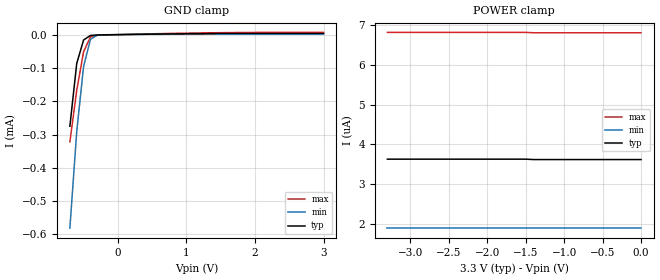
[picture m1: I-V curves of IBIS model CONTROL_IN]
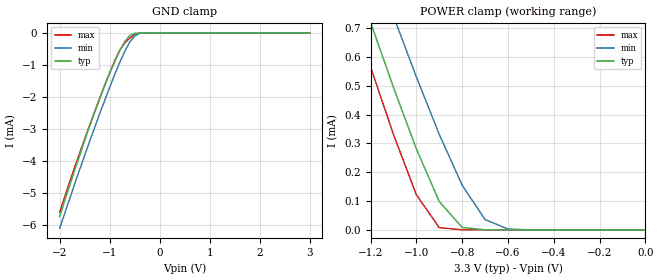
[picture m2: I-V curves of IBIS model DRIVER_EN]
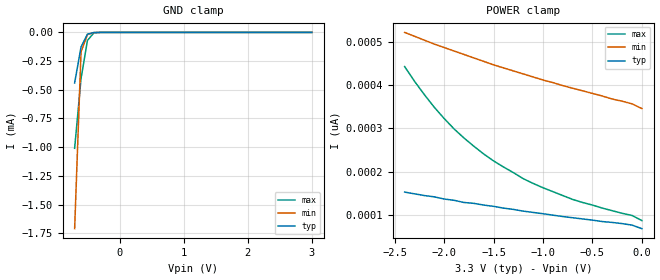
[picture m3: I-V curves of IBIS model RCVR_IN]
|   Texas Instruments Incorporated
|   Data Transmissions Products
|   IBIS Model for SN65LVDS122
|   16D SOIC Package
[IBIS Ver]   3.2
[Comment char]   |_char
[File name]   lvds122.ibs
[File Rev]   3.0
[Date]   22Sep03
[Source]   File originated at Texas Instruments Incorporated.
   Data Transmission Products Group.
[Notes]
[Disclaimer]
(C) Copyright Texas Instruments Incorporated 2002
   All rights reserved
  Texas Instruments Incorporated hereby grants the user of this IBIS
model a non-exclusive, nontransferable license to use this IBIS model
under the following terms.  Before using this IBIS model, the user
should read this license.  If the user does not accept these terms,
the IBIS model should be returned to Texas Instruments within 30 days.
  The user is granted this license only to use the IBIS model and
is not granted rights to sell, load, rent, lease or license the IBIS
model in whole or in part, or in modified form to anyone other than
user.  User may modify the IBIS model to suit its specific applications
but rights to derivative works and such modifications shall belong to
Texas Instruments.
  This IBIS model is provided on an "AS IS" basis and Texas Instruments
makes absolutely no warranty with respect to the information contained
herein.  TEXAS INSTRUMENTS DISCLAIMS AND CUSTOMER WAIVES ALL WARRANTIES,
EXPRESS OR IMPLIED, INCLUDING WARRANTIES OF MERCHANTABILITY OR FITNESS
FOR A PARTICULAR PURPOSE. The entire risk as to quality and performance
is with the Customer. ACCORDINGLY, IN NO EVENT SHALL THE COMPANY BE LIABLE
FOR ANY DAMAGES, WHETHER IN CONTRACT OR TORT,INCLUDING ANY LOST PROFITS
OR OTHER INCIDENTAL, CONSEQUENTIAL, EXEMPLARY, OR PUNITIVE DAMAGES ARISING
OUT OF THE USE OR APPLICATION OF THE IBIS model provided in this package.
Further, Texas Instruments reserves the right to discontinue or make changes
without notice to any product herein to improve reliability, function, or
design. Texas Instruments does not convey any license under patent rights
or any other intellectual property rights, including those of third parties.
Contact Texas Instruments at ATTN:DATA TRANSMISSIONS
[Copyright]   Copyright 2002, Texas Instruments, All Rights Reserved
[Component]   LVDS122D
[Manufacturer]  Texas Instruments Incorporated
[Package]
|   typ   min   max
R_pkg   0.035   0.030   0.040
L_pkg   2.181nH   1.231nH   3.257nH
C_pkg   0.322pF   0.163pF   0.546pF
[Pin]   signal_name   model_name   R_pin   L_pin   C_pin
1   1B   RCVR_IN   0.040   3.251n   0.546p
2   1A   RCVR_IN   0.039   2.561n   0.393p
3   S0   CONTROL_IN   0.030   1.681n   0.186p
4   1DE   DRIVER_EN   0.030   1.231n   0.163p
5   S1   CONTROL_IN   0.030   1.231n   0.163p
6   2A   RCVR_IN   0.030   1.681n   0.186p
7   2B   RCVR_IN   0.039   2.564n   0.393p
8   GND   GND   0.040   3.257n   0.545p
9   GND   GND   0.040   3.247n   0.546p
10   2Y   DRVR_OUT   0.039   2.558n   0.394p
11   2Z   DRVR_OUT   0.030   1.681n   0.187p
12   2DE   DRIVER_EN   0.030   1.231n   0.163p
13   1Z   DRVR_OUT   0.030   1.231n   0.163p
14   1Y   DRVR_OUT   0.030   1.681n   0.187p
15   VCC   POWER   0.039   2.558n   0.394p
16   VCC   POWER   0.040   3.246n   0.546p
[Diff_pin]   inv_pin   vdiff   tdelay_typ   tdelay_min   tdelay_max
| The 'xY' pin is Diff_pin and the 'xZ' pin is the inv_pin
2   1   0.100   0 0 0
6   7   0.100   0 0 0
14   13   NA   0 0 0
10   11   NA   0 0 0
| Models and submodels in the file (4): CONTROL_IN (Input), DRIVER_EN (Input), RCVR_IN (Input), DRVR_OUT (Output)
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|   Control Input Model
[Model]   CONTROL_IN
Model_type   Input
|Signals   S0,S1
Vinh = 2.0
Vinl = 0.8
|   typ   min   max
C_comp   3.0pF   2.2pF   3.9pF
|   typ   min   max
[Temperature Range]   25.0   85   -40
[Voltage range]   3.3V   3.0V   3.6V
[GND_clamp]
|   Voltage   I(typ)   I(min)   I(max)
-700mV    -275uA     -581uA     -322uA
-600mV    -86.4uA    -291uA     -167uA
-500mV    -16.1uA    -95.3uA    -51.3uA
-400mV    -2.4uA     -14.1uA    -6.64uA
-300mV    -1.09uA    -1.48uA    -1.92uA
-200mV    -688nA     -442nA     -1.19uA
1.3V      3uA        1.64uA     5.35uA
3V        3.62uA     1.9uA      6.79uA
[Power_clamp]
| Note that the[POWER_clamp]voltage table is referenced to Vcc
| and is calculated using Vtable=Vcc - Vmeasured.
|   Voltage   I(typ)   I(min)   I(max)
-3.3V     3.63uA     1.9uA      6.81uA
-1.5V     3.63uA     1.9uA      6.81uA
-1.4V     3.62uA     1.9uA      6.8uA
0V        3.62uA     1.9uA      6.8uA
|   Driver Enable Model
[Model]   DRIVER_EN
Model_type   Input
|Signals   1DE,2DE
Vinh = 2.0
Vinl = 0.8
|   typ   min   max
C_comp   3.0pF   2.2pF   3.9pF
|   typ   min   max
[Temperature Range]   25.0   85   -40
[Voltage range]   3.3V   3.0V   3.6V
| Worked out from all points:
|   GND clamp passes 1 mA (typ) near -0.93 V on its own axis
|   POWER clamp passes 1 mA (typ) near -1.32 V on its own axis
[GND_clamp]
|   Voltage   I(typ)   I(min)   I(max)
-2V       -5.73mA    -6.09mA    -5.6mA
-1.8V     -4.76mA    -5.17mA    -4.64mA
-1.5V     -3.35mA    -3.82mA    -3.31mA
-1.1V     -1.63mA    -2.11mA    -1.64mA
-900mV    -894uA     -1.3mA     -877uA
-800mV    -563uA     -927uA     -543uA
-700mV    -275uA     -581uA     -320uA
-600mV    -85.4uA    -290uA     -165uA
-500mV    -15.1uA    -94.7uA    -49.8uA
-400mV    -1.56uA    -13.7uA    -5.11uA
-300mV    -610nA     -1.28uA    -938nA
3V        -141nA     249pA      -354nA
[Power_clamp]
| Note that the[POWER_clamp]voltage table is referenced to Vcc
| and is calculated using Vtable=Vcc - Vmeasured.
|   Voltage   I(typ)   I(min)   I(max)
-2.4V     3.62mA     3.7mA      3.61mA
-1.3V     952uA      1.18mA     808uA
-1.2V     720uA      958uA      565uA
-1.1V     494uA      741uA      331uA
-1V       281uA      530uA      122uA
-900mV    98.5uA     331uA      7.98uA
-800mV    8.69uA     155uA      648nA
-700mV    589nA      36.1uA     514nA
-600mV    339nA      3.16uA     438nA
-500mV    276nA      371nA      362nA
0V        44.3pA     249pA      67.9pA
|   Receiver Input Model
[Model]   RCVR_IN
Model_type   Input
|Signals   1A,1B,2A,2B
Vinh = 1.4
Vinl = 1.0
|   typ   min   max
C_comp   1.0pF   0.5p   1.4p
|   typ   min   max
[Temperature Range]   25.0   85   -40
[Voltage range]   3.3V   3.0V   3.6V
[GND_clamp]
|   Voltage   I(typ)   I(min)   I(max)
-700mV    -441uA     -1.71mA    -1.01mA
-600mV    -126uA     -168uA     -401uA
-500mV    -15.3uA    -19.6uA    -70.1uA
-400mV    -897nA     -1.88uA    -3.96uA
-300mV    -32.9nA    -145nA     -91.1nA
3V        55.9pA     346pA      58.2pA
[Power_clamp]
| Note that the[POWER_clamp]voltage table is referenced to Vcc
| and is calculated using Vtable=Vcc - Vmeasured.
|   Voltage   I(typ)   I(min)   I(max)
-2.4V     153pA      522pA      443pA
-2.2V     145pA      504pA      378pA
-2V       137pA      487pA      323pA
-1.8V     129pA      471pA      278pA
-1.6V     123pA      455pA      241pA
-1.5V     120pA      447pA      225pA
-1.2V     109pA      426pA      184pA
-1V       103pA      412pA      163pA
-700mV    93.7pA     393pA      136pA
-200mV    80.2pA     363pA      104pA
-100mV    76.7pA     357pA      99pA
0V        68.5pA     346pA      87.2pA
